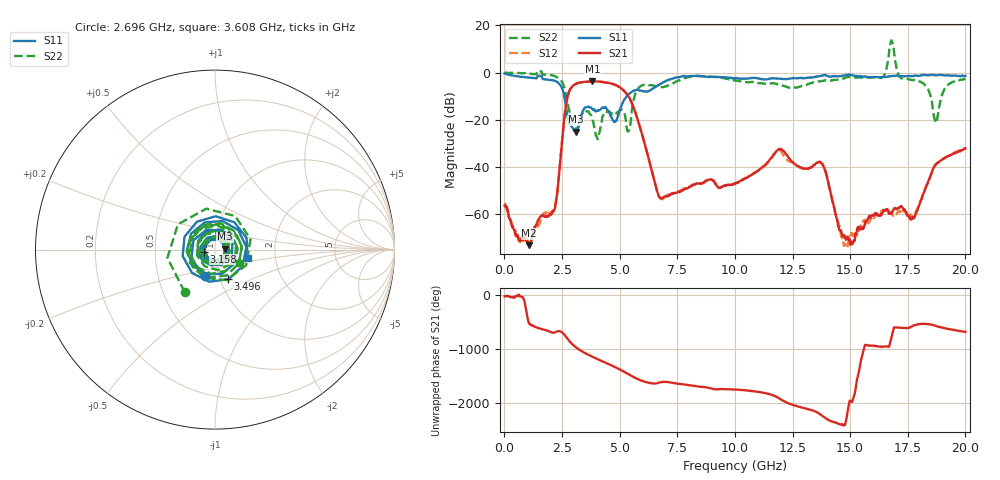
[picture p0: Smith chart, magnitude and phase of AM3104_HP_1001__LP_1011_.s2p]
!Created with skrf (http://scikit-rf.org).
# Hz S RI R 50.0
!freq ReS11 ImS11 ReS21 ImS21 ReS12 ImS12 ReS22 ImS22
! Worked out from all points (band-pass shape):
!   1601 points, 10 MHz to 20 GHz, reference 50 ohm
!   highest |S21| = -3.70 dB at 3.821 GHz (marker M1); lowest = -73.3 dB at 1.072 GHz (marker M2)
!   |S21| within 3 dB of the highest: 2.878 GHz to 5.076 GHz (2.198 GHz wide, 55.3 % of centre)
!   lowest |S11| = -25.1 dB at 3.096 GHz (marker M3), VSWR 1.12, Z = 55.9 + j0.552 ohm
!   |S11| at or under -10 dB: 2.597 GHz to 5.309 GHz (2.712 GHz wide, 68.6 % of centre)
!   |S22| runs from -28.2 to 13.6 dB; largest |S21 - S12| = 0.054
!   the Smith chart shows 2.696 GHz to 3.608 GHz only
!   S11 on the Smith chart (normalised r, x): 2.696 GHz: 0.86, -0.25; 3.158 GHz: 0.88, -0.02; 3.496 GHz: 1.09, -0.37; 3.608 GHz: 1.44, -0.13
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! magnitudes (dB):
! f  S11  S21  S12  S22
! 10 MHz  -0.4  -56.4  -55.4  -0.1
! 1.072 GHz  -2.1  -73.3  -71.1  -0.4
! 2.196 GHz  -3.5  -57.4  -56.9  -1.6
! 2.696 GHz  -16.1  -12.5  -12.5  -10.7
! 3.096 GHz  -25.1  -4.8  -4.8  -23.8
! 3.158 GHz  -24.1  -4.5  -4.6  -24.0
! 3.346 GHz  -18.0  -4.1  -4.2  -18.5
! 3.496 GHz  -14.8  -3.9  -4.0  -16.0
! 3.608 GHz  -14.5  -3.8  -3.9  -16.4
! 3.821 GHz  -15.4  -3.7  -3.7  -20.1
! 5.395 GHz  -9.2  -10.3  -10.3  -24.8
! 5.795 GHz  -7.3  -20.3  -20.3  -6.8
! 6.682 GHz  -5.3  -51.8  -52.1  -6.0
! 10.01 GHz  -2.5  -47.1  -47.3  -3.4
! 11.93 GHz  -2.5  -32.4  -32.7  -5.2
! 13.34 GHz  -2.1  -40.0  -40.0  -4.4
! 13.87 GHz  -1.1  -40.2  -39.9  -3.4
! 14.82 GHz  -1.0  -70.9  -73.2  -2.1
! 16.68 GHz  -1.6  -59.6  -58.7  7.2
! 17.73 GHz  -1.4  -62.0  -61.5  -3.2
! 18.71 GHz  -1.2  -38.9  -39.1  -21.1
! 20 GHz  -1.4  -32.2  -32.1  -2.7
